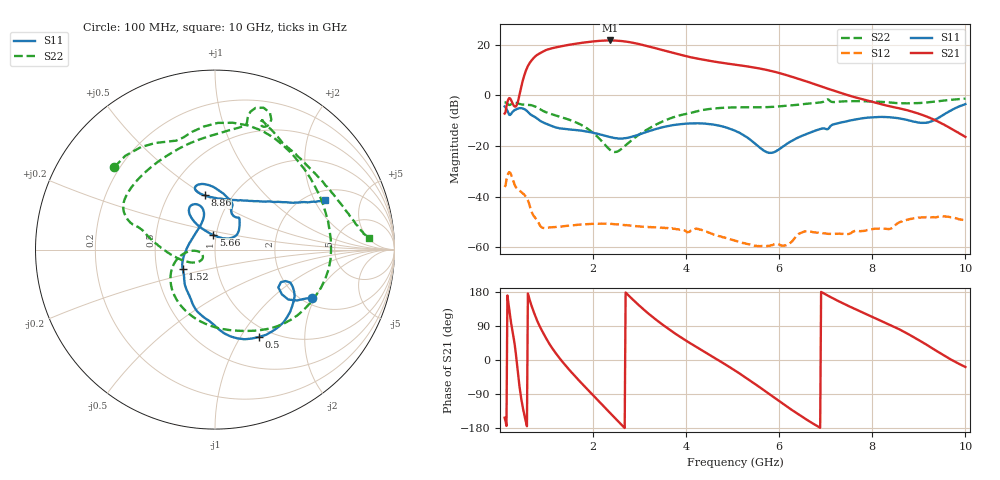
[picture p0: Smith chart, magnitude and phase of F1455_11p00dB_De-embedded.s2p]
! Integrated Device Technology
! Corporate Headquarters
! 6024 Silver Creek Valley Road
! San Jose, CA 95138  USA
! Phone:  1-408-284-8200
! Toll Free:  1-800-223-1366
! Webpage:  http://www.idt.com/
! Timing and RF Division
! 515 Groton Road, Suite 102
! Westford, MA 01886-6024
! Device:  F1455
! Description: 6-bit 0.5 dB Transmit Variable Gain Amplifier
! Frequency:  1400.0 -  2300.00 MHz
! Package:  6x6 mm Thin QFN Plastic Package: 28 pin
! State:  22
! Atten State:  11.0 dB
! Voltage:  +5.00 Volts
! Current:  217.674 mA
! Data:  The device was measured on a the F1455 evaluation board which has
!  individual transmission lines to the RF pins.  Data was collected
!  using a calibrated network analyzer.  The evaluation board was
!  de-embedded using a TRL calibration technique.
!  The reference plane is the edge of the package pin.
!  Pin  1 = CSb
!  Pin  2 = DATA
!  Pin  3 = CLK
!  Pin  4 = RSET
!  Pin  5 = GND
!  Pin  6 = RFIN  = Port 1
!  Pin  7 = GND
!  Pin  8 = NC
!  Pin  9 = NC
!  Pin 10 = NC
!  Pin 11 = NC
!  Pin 12 = NC
!  Pin 13 = NC
!  Pin 14 = /STBY
!  Pin 15 = GND
!  Pin 16 = RFOUT  = Port 2
!  Pin 17 = GND
!  Pin 18 = NC
!  Pin 19 = NC
!  Pin 20 = NC
!  Pin 21 = GND
!  Pin 22 = NC
!  Pin 23 = GND
!  Pin 24 = NC
!  Pin 25 = NC
!  Pin 26 = NC
!  Pin 27 = GND
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# GHz S dB R 50
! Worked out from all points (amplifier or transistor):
!   496 points, 100 MHz to 10 GHz, reference 50 ohm
!   highest |S21| = 21.7 dB at 2.36 GHz (marker M1)
!   |S21| within 3 dB of that: 1.14 GHz to 3.329 GHz (2.189 GHz wide, 98 % of centre)
!   unconditionally stable (mu >= 1): start of sweep to end of sweep
!   at 1.74 GHz: K = 14.69, MAG = 21.2 dB, |S12| = -51.0 dB
!   at 5.06 GHz: K = 59.66, MAG = 14.1 dB, |S12| = -57.6 dB
!   at 10 GHz: K = 138.50, MAG = -7.9 dB, |S12| = -49.5 dB
!   S11 on the Smith chart (normalised r, x): 100 MHz: 2.23, -1.89; 500 MHz: 0.87, -1.21; 1.52 GHz: 0.68, -0.16; 5.66 GHz: 0.97, +0.16; 8.86 GHz: 0.75, +0.50; 10 GHz: 2.44, +2.43
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0.1  -4.40 -26.6  -7.21 -152.2  -36.19 45.1  -2.79 140.7
0.38  -5.29 -39.8  -2.89 -27.0  -37.06 -113.0  -3.18 56.8
0.5  -5.27 -63.3  6.48 -131.0  -38.89 -150.9  -3.66 27.4
0.68  -7.83 -93.2  13.83 142.6  -46.00 147.4  -3.94 -14.9
0.8  -9.17 -108.4  16.00 103.6  -49.42 131.7  -4.80 -42.9
0.94  -10.82 -120.8  17.46 68.9  -52.44 124.3  -6.29 -69.2
1.22  -12.79 -138.8  19.03 14.5  -52.01 94.4  -8.08 -108.0
1.52  -13.54 -148.8  20.08 -30.2  -51.47 64.8  -9.86 -138.8
1.76  -13.99 -156.2  20.76 -62.1  -51.03 46.2  -11.82 -157.6
2.06  -15.01 -168.3  21.42 -100.5  -50.74 25.9  -15.77 -174.4
2.36  -16.46 170.8  21.70 -139.0  -50.82 8.1  -21.47 -169.6
2.56  -17.06 151.3  21.55 -164.4  -51.07 -2.5  -21.86 -146.9
2.76  -16.74 131.7  21.10 170.8  -51.39 -11.6  -18.82 -143.7
3.06  -15.04 112.4  19.95 136.3  -51.90 -23.1  -14.70 -160.2
3.4  -13.07 106.5  18.35 102.0  -52.21 -35.0  -11.17 -178.6
4.08  -11.12 114.7  15.13 44.8  -53.87 -53.6  -7.01 163.6
5.06  -14.06 126.5  12.11 -28.6  -57.55 -93.9  -4.75 148.2
5.66  -21.75 96.6  10.32 -78.8  -59.60 -93.9  -4.69 124.0
6.7  -14.49 43.6  4.79 -165.8  -53.95 -135.9  -3.14 78.3
8.36  -8.65 106.8  -4.29 93.6  -52.88 163.1  -2.79 62.2
8.86  -10.21 100.9  -6.47 62.4  -48.72 146.2  -3.16 42.7
10  -3.47 24.1  -16.42 -18.5  -49.47 72.0  -1.29 4.5
